FUNCTION_BLOCK FB101
TITLE =
VERSION : 0.1


VAR
  F_GAS_BU : "GAS_BU";	//Ovládání hoøáku
  F_TIGHTN : "TIGHTN";	//Test tìsnosti
  F_PRE_PURGE : "PRE_PURGE";	//Provìtrávání
  F_AIRD_GAS : "AIRD";	//Test polohy klapy plynu
  F_AIRD_AIR : "AIRD";	//Test polohy klapy vzduchu
  F_POS_CH : "POS_CH";	//Test funkce regulaèních klap
  F_IGNTR : "IGNTR";	//Zapalovací hoøák
  tBIT : BOOL ;
END_VAR
VAR_TEMP
  tB : BOOL ;
END_VAR
BEGIN
NETWORK
TITLE =Uvolnìní bezp.relé napájení
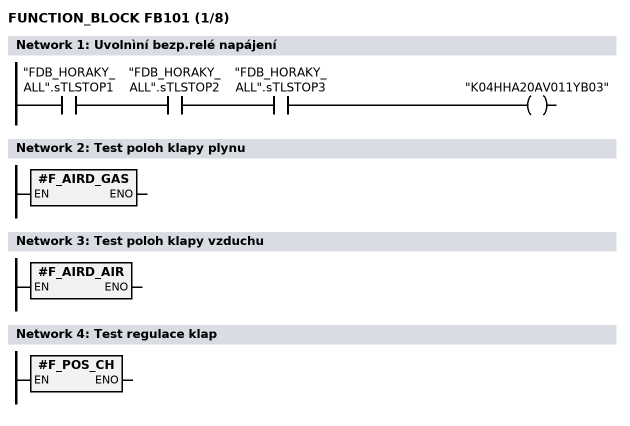
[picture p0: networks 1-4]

      A     "FDB_HORAKY_ALL".sTLSTOP1;
      A     "FDB_HORAKY_ALL".sTLSTOP2;
      A     "FDB_HORAKY_ALL".sTLSTOP3;
      =     "K04HHA20AV011YB03";
NETWORK
TITLE =Test poloh klapy plynu

      CALL #F_AIRD_GAS ;
      NOP   0;
NETWORK
TITLE =Test poloh klapy vzduchu

      CALL #F_AIRD_AIR ;
      NOP   0;
NETWORK
TITLE =Test regulace klap

      CALL #F_POS_CH ;
      NOP   0;
NETWORK
TITLE =Diagnostika klap plynu a vzduchu
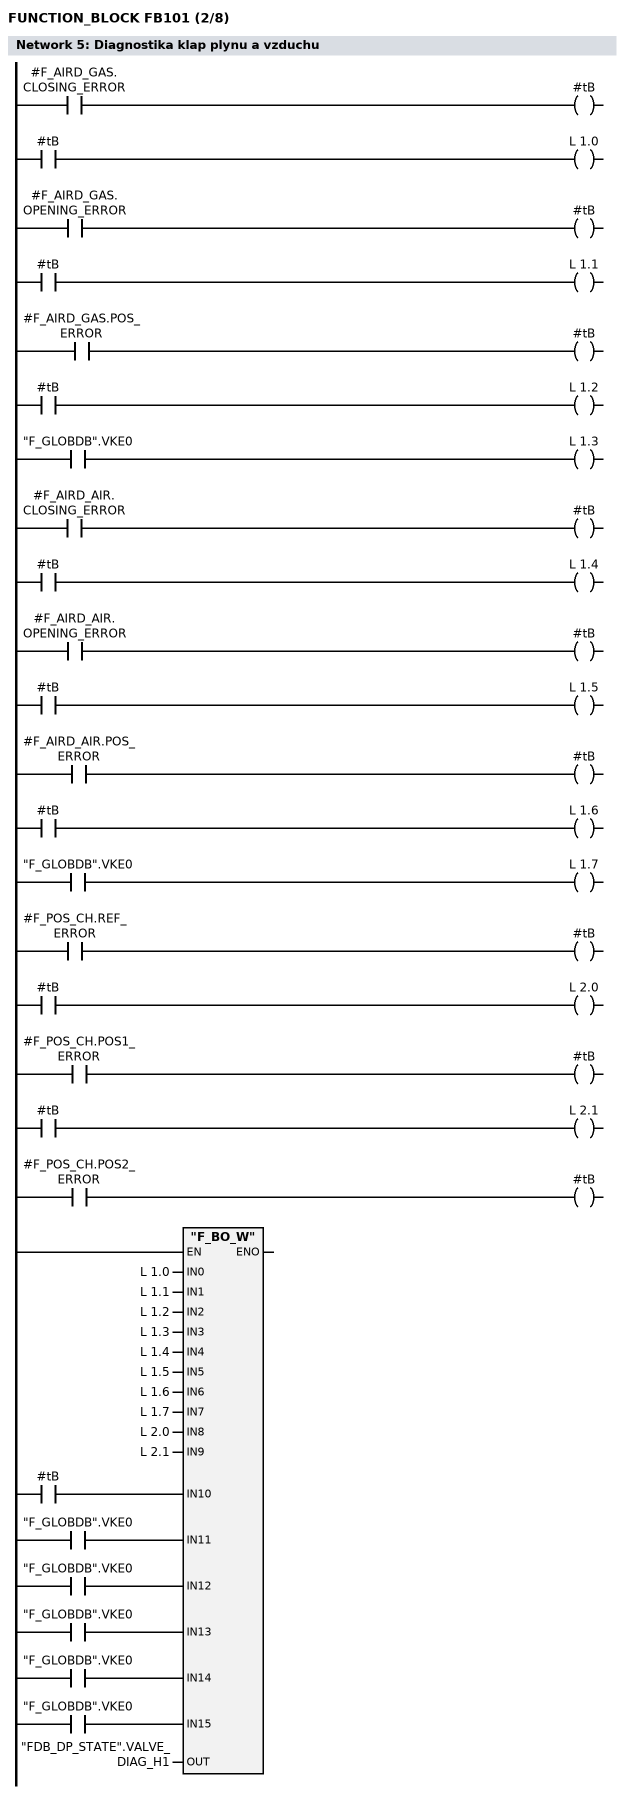
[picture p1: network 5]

      A     #F_AIRD_GAS.CLOSING_ERROR;
      =     #tB;
      A     #tB;
      =     L      1.0;
      BLD   103;
      A     #F_AIRD_GAS.OPENING_ERROR;
      =     #tB;
      A     #tB;
      =     L      1.1;
      BLD   103;
      A     #F_AIRD_GAS.POS_ERROR;
      =     #tB;
      A     #tB;
      =     L      1.2;
      BLD   103;
      A     "F_GLOBDB".VKE0;
      =     L      1.3;
      BLD   103;
      A     #F_AIRD_AIR.CLOSING_ERROR;
      =     #tB;
      A     #tB;
      =     L      1.4;
      BLD   103;
      A     #F_AIRD_AIR.OPENING_ERROR;
      =     #tB;
      A     #tB;
      =     L      1.5;
      BLD   103;
      A     #F_AIRD_AIR.POS_ERROR;
      =     #tB;
      A     #tB;
      =     L      1.6;
      BLD   103;
      A     "F_GLOBDB".VKE0;
      =     L      1.7;
      BLD   103;
      A     #F_POS_CH.REF_ERROR;
      =     #tB;
      A     #tB;
      =     L      2.0;
      BLD   103;
      A     #F_POS_CH.POS1_ERROR;
      =     #tB;
      A     #tB;
      =     L      2.1;
      BLD   103;
      A     #F_POS_CH.POS2_ERROR;
      =     #tB;
      A     #tB;
      =     L      2.2;
      BLD   103;
      A     "F_GLOBDB".VKE0;
      =     L      2.3;
      BLD   103;
      A     "F_GLOBDB".VKE0;
      =     L      2.4;
      BLD   103;
      A     "F_GLOBDB".VKE0;
      =     L      2.5;
      BLD   103;
      A     "F_GLOBDB".VKE0;
      =     L      2.6;
      BLD   103;
      A     "F_GLOBDB".VKE0;
      =     L      2.7;
      BLD   103;
      CALL "F_BO_W" (
           IN0                      := L      1.0,
           IN1                      := L      1.1,
           IN2                      := L      1.2,
           IN3                      := L      1.3,
           IN4                      := L      1.4,
           IN5                      := L      1.5,
           IN6                      := L      1.6,
           IN7                      := L      1.7,
           IN8                      := L      2.0,
           IN9                      := L      2.1,
           IN10                     := L      2.2,
           IN11                     := L      2.3,
           IN12                     := L      2.4,
           IN13                     := L      2.5,
           IN14                     := L      2.6,
           IN15                     := L      2.7,
           OUT                      := "FDB_DP_STATE".VALVE_DIAG_H1);
      NOP   0;
NETWORK
TITLE =Provìtrávání
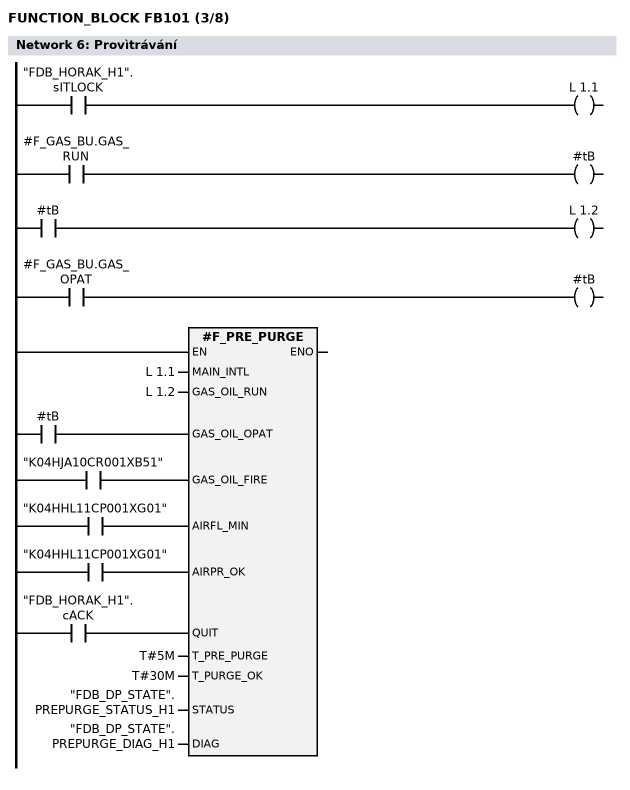
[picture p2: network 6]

      A     "FDB_HORAK_H1".sITLOCK;
      =     L      1.1;
      BLD   103;
      A     #F_GAS_BU.GAS_RUN;
      =     #tB;
      A     #tB;
      =     L      1.2;
      BLD   103;
      A     #F_GAS_BU.GAS_OPAT;
      =     #tB;
      A     #tB;
      =     L      1.3;
      BLD   103;
      A     "K04HJA10CR001XB51";
      =     L      1.4;
      BLD   103;
      A     "K04HHL11CP001XG01";
      =     L      1.6;
      BLD   103;
      A     "K04HHL11CP001XG01";
      =     L      1.7;
      BLD   103;
      A     "FDB_HORAK_H1".cACK;
      =     L      2.3;
      BLD   103;
      CALL #F_PRE_PURGE (
           MAIN_INTL                := L      1.1,
           GAS_OIL_RUN              := L      1.2,
           GAS_OIL_OPAT             := L      1.3,
           GAS_OIL_FIRE             := L      1.4,
           AIRFL_MIN                := L      1.6,
           AIRPR_OK                 := L      1.7,
           QUIT                     := L      2.3,
           T_PRE_PURGE              := T#5M,
           T_PURGE_OK               := T#30M,
           STATUS                   := "FDB_DP_STATE".PREPURGE_STATUS_H1,
           DIAG                     := "FDB_DP_STATE".PREPURGE_DIAG_H1);
      NOP   0;
NETWORK
TITLE =Test tìsnosti
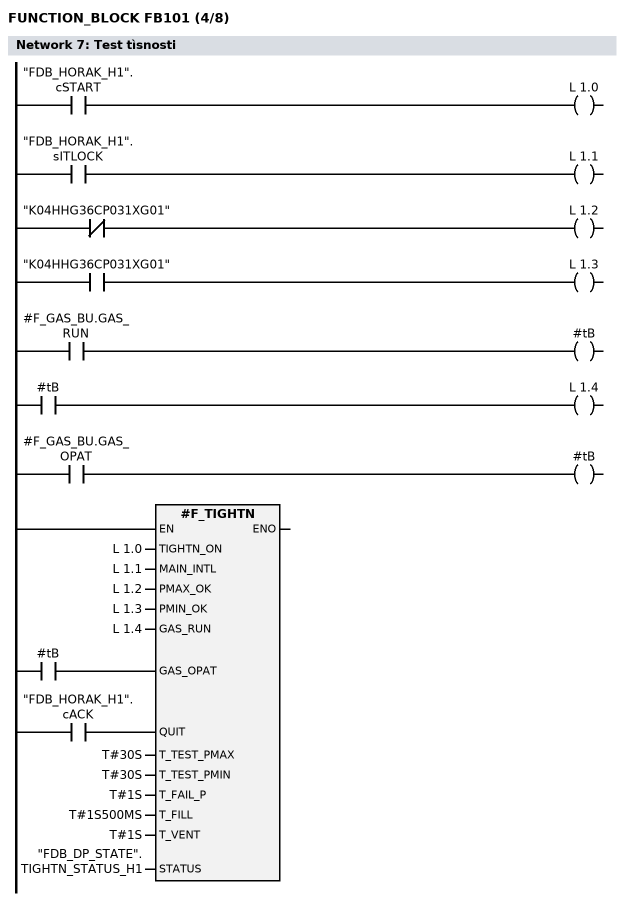
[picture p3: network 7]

      A     "FDB_HORAK_H1".cSTART;
      =     L      1.0;
      BLD   103;
      A     "FDB_HORAK_H1".sITLOCK;
      =     L      1.1;
      BLD   103;
      AN    "K04HHG36CP031XG01";
      =     L      1.2;
      BLD   103;
      A     "K04HHG36CP031XG01";
      =     L      1.3;
      BLD   103;
      A     #F_GAS_BU.GAS_RUN;
      =     #tB;
      A     #tB;
      =     L      1.4;
      BLD   103;
      A     #F_GAS_BU.GAS_OPAT;
      =     #tB;
      A     #tB;
      =     L      1.5;
      BLD   103;
      A     "FDB_HORAK_H1".cACK;
      =     L      1.6;
      BLD   103;
      CALL #F_TIGHTN (
           TIGHTN_ON                := L      1.0,
           MAIN_INTL                := L      1.1,
           PMAX_OK                  := L      1.2,
           PMIN_OK                  := L      1.3,
           GAS_RUN                  := L      1.4,
           GAS_OPAT                 := L      1.5,
           QUIT                     := L      1.6,
           T_TEST_PMAX              := T#30S,
           T_TEST_PMIN              := T#30S,
           T_FAIL_P                 := T#1S,
           T_FILL                   := T#1S500MS,
           T_VENT                   := T#1S,
           STATUS                   := "FDB_DP_STATE".TIGHTN_STATUS_H1);
      NOP   0;
NETWORK
TITLE =Diagnostika testu tìsnosti
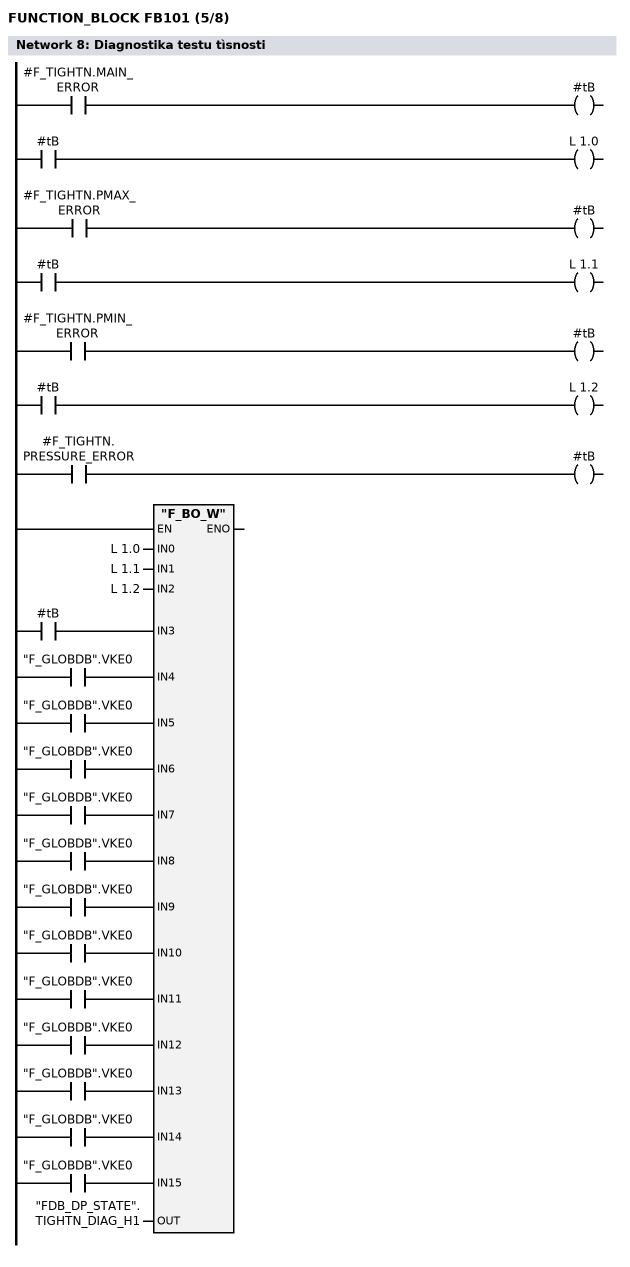
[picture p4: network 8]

      A     #F_TIGHTN.MAIN_ERROR;
      =     #tB;
      A     #tB;
      =     L      1.0;
      BLD   103;
      A     #F_TIGHTN.PMAX_ERROR;
      =     #tB;
      A     #tB;
      =     L      1.1;
      BLD   103;
      A     #F_TIGHTN.PMIN_ERROR;
      =     #tB;
      A     #tB;
      =     L      1.2;
      BLD   103;
      A     #F_TIGHTN.PRESSURE_ERROR;
      =     #tB;
      A     #tB;
      =     L      1.3;
      BLD   103;
      A     "F_GLOBDB".VKE0;
      =     L      1.4;
      BLD   103;
      A     "F_GLOBDB".VKE0;
      =     L      1.5;
      BLD   103;
      A     "F_GLOBDB".VKE0;
      =     L      1.6;
      BLD   103;
      A     "F_GLOBDB".VKE0;
      =     L      1.7;
      BLD   103;
      A     "F_GLOBDB".VKE0;
      =     L      2.0;
      BLD   103;
      A     "F_GLOBDB".VKE0;
      =     L      2.1;
      BLD   103;
      A     "F_GLOBDB".VKE0;
      =     L      2.2;
      BLD   103;
      A     "F_GLOBDB".VKE0;
      =     L      2.3;
      BLD   103;
      A     "F_GLOBDB".VKE0;
      =     L      2.4;
      BLD   103;
      A     "F_GLOBDB".VKE0;
      =     L      2.5;
      BLD   103;
      A     "F_GLOBDB".VKE0;
      =     L      2.6;
      BLD   103;
      A     "F_GLOBDB".VKE0;
      =     L      2.7;
      BLD   103;
      CALL "F_BO_W" (
           IN0                      := L      1.0,
           IN1                      := L      1.1,
           IN2                      := L      1.2,
           IN3                      := L      1.3,
           IN4                      := L      1.4,
           IN5                      := L      1.5,
           IN6                      := L      1.6,
           IN7                      := L      1.7,
           IN8                      := L      2.0,
           IN9                      := L      2.1,
           IN10                     := L      2.2,
           IN11                     := L      2.3,
           IN12                     := L      2.4,
           IN13                     := L      2.5,
           IN14                     := L      2.6,
           IN15                     := L      2.7,
           OUT                      := "FDB_DP_STATE".TIGHTN_DIAG_H1);
      NOP   0;
NETWORK
TITLE =Hlavní hoøák
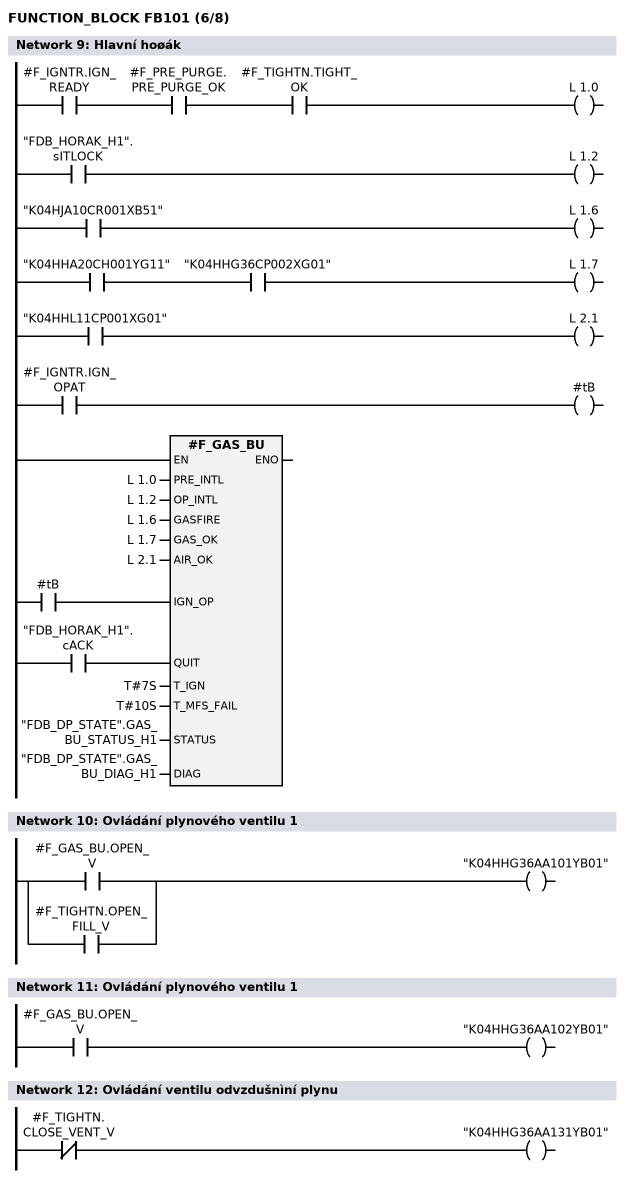
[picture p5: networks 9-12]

      A     #F_IGNTR.IGN_READY;
      A     #F_PRE_PURGE.PRE_PURGE_OK;
      A     #F_TIGHTN.TIGHT_OK;
      =     L      1.0;
      BLD   103;
      A     "FDB_HORAK_H1".sITLOCK;
      =     L      1.2;
      BLD   103;
      A     "K04HJA10CR001XB51";
      =     L      1.6;
      BLD   103;
      A     "K04HHA20CH001YG11";
      A     "K04HHG36CP002XG01";
      =     L      1.7;
      BLD   103;
      A     "K04HHL11CP001XG01";
      =     L      2.1;
      BLD   103;
      A     #F_IGNTR.IGN_OPAT;
      =     #tB;
      A     #tB;
      =     L      2.2;
      BLD   103;
      A     "FDB_HORAK_H1".cACK;
      =     L      2.4;
      BLD   103;
      CALL #F_GAS_BU (
           PRE_INTL                 := L      1.0,
           OP_INTL                  := L      1.2,
           GASFIRE                  := L      1.6,
           GAS_OK                   := L      1.7,
           AIR_OK                   := L      2.1,
           IGN_OP                   := L      2.2,
           QUIT                     := L      2.4,
           T_IGN                    := T#7S,
           T_MFS_FAIL               := T#10S,
           STATUS                   := "FDB_DP_STATE".GAS_BU_STATUS_H1,
           DIAG                     := "FDB_DP_STATE".GAS_BU_DIAG_H1);
      NOP   0;
NETWORK
TITLE =Ovládání plynového ventilu 1

      O     #F_GAS_BU.OPEN_V;
      O     #F_TIGHTN.OPEN_FILL_V;
      =     "K04HHG36AA101YB01";
NETWORK
TITLE =Ovládání plynového ventilu 1

      A     #F_GAS_BU.OPEN_V;
      =     "K04HHG36AA102YB01";
NETWORK
TITLE =Ovládání ventilu odvzdušnìní plynu

      AN    #F_TIGHTN.CLOSE_VENT_V;
      =     "K04HHG36AA131YB01";
NETWORK
TITLE =Zapalovací hoøák
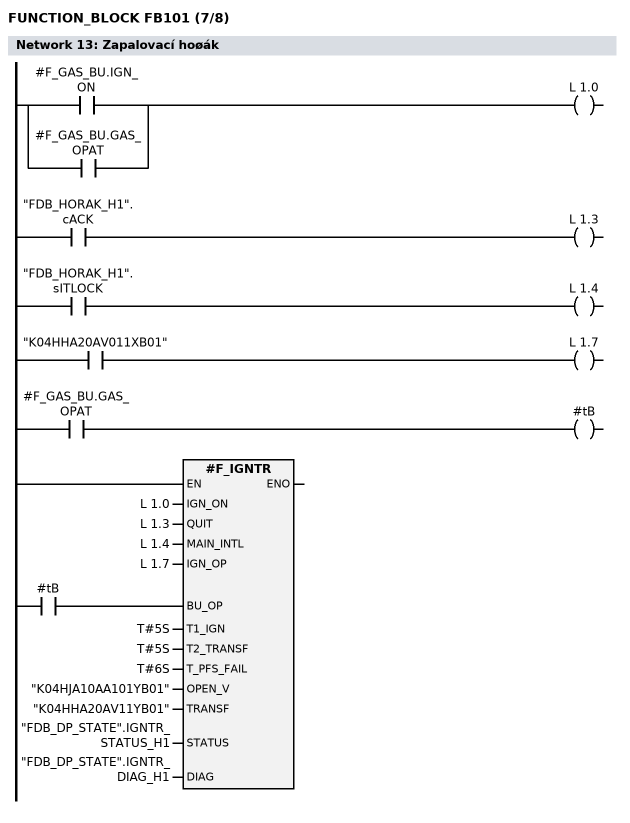
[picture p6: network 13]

      A(    ;
      O     #F_GAS_BU.IGN_ON;
      O     #F_GAS_BU.GAS_OPAT;
      )     ;
      =     L      1.0;
      BLD   103;
      A     "FDB_HORAK_H1".cACK;
      =     L      1.3;
      BLD   103;
      A     "FDB_HORAK_H1".sITLOCK;
      =     L      1.4;
      BLD   103;
      A     "K04HHA20AV011XB01";
      =     L      1.7;
      BLD   103;
      A     #F_GAS_BU.GAS_OPAT;
      =     #tB;
      A     #tB;
      =     L      2.2;
      BLD   103;
      CALL #F_IGNTR (
           IGN_ON                   := L      1.0,
           QUIT                     := L      1.3,
           MAIN_INTL                := L      1.4,
           IGN_OP                   := L      1.7,
           BU_OP                    := L      2.2,
           T1_IGN                   := T#5S,
           T2_TRANSF                := T#5S,
           T_PFS_FAIL               := T#6S,
           OPEN_V                   := "K04HJA10AA101YB01",
           TRANSF                   := "K04HHA20AV11YB01",
           STATUS                   := "FDB_DP_STATE".IGNTR_STATUS_H1,
           DIAG                     := "FDB_DP_STATE".IGNTR_DIAG_H1);
      NOP   0;
NETWORK
TITLE =Vyhodnocení nutnosti kvitace
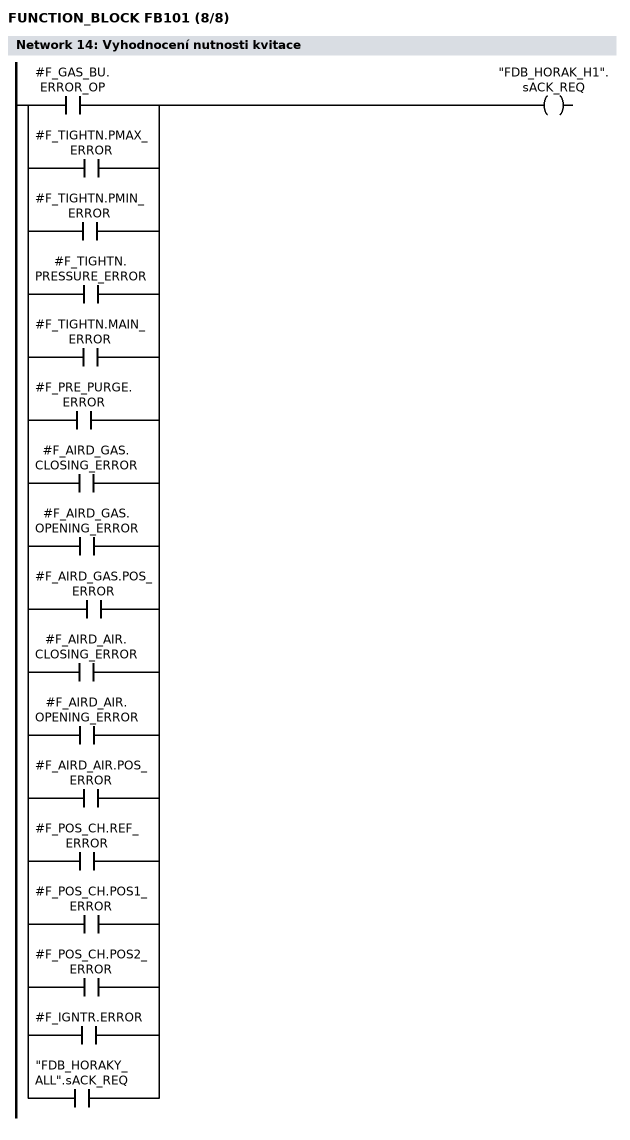
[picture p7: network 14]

      O     #F_GAS_BU.ERROR_OP;
      O     #F_TIGHTN.PMAX_ERROR;
      O     #F_TIGHTN.PMIN_ERROR;
      O     #F_TIGHTN.PRESSURE_ERROR;
      O     #F_TIGHTN.MAIN_ERROR;
      O     #F_PRE_PURGE.ERROR;
      O     #F_AIRD_GAS.CLOSING_ERROR;
      O     #F_AIRD_GAS.OPENING_ERROR;
      O     #F_AIRD_GAS.POS_ERROR;
      O     #F_AIRD_AIR.CLOSING_ERROR;
      O     #F_AIRD_AIR.OPENING_ERROR;
      O     #F_AIRD_AIR.POS_ERROR;
      O     #F_POS_CH.REF_ERROR;
      O     #F_POS_CH.POS1_ERROR;
      O     #F_POS_CH.POS2_ERROR;
      O     #F_IGNTR.ERROR;
      O     "FDB_HORAKY_ALL".sACK_REQ;
      =     "FDB_HORAK_H1".sACK_REQ;
END_FUNCTION_BLOCK

